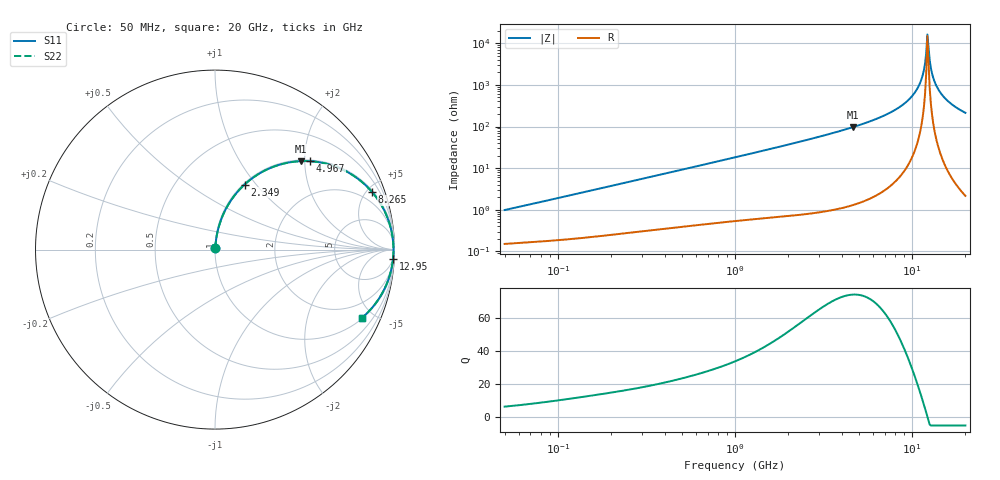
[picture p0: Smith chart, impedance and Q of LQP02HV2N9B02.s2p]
!Murata Part Number: LQP02HV2N9B02
!These Parameters are Measured in Series Mode Connection
!  o--[Z]--o
!Port1  Port2
!  o-------o
!Freq. Start=50[MHz] Stop=20[GHz], 401[Steps]
# Hz S RI R 50
!Freq.(Hz) S11(Real) S11(Imag) S21(Real) S21(Imag) S12(Real) S12(Imag) S22(Real) S22(Imag)
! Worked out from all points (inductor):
!   401 points, 50 MHz to 20 GHz, reference 50 ohm
!   read as one part in series: L = 3.08 nH near 51.52 MHz
!   highest Q = 74.4 at 4.608 GHz (marker M1), where L = 3.32 nH
!   self-resonance near 12.2 GHz
!   S11 on the Smith chart (normalised r, x): 50 MHz: 1.00, +0.02; 2.349 GHz: 1.02, +0.87; 4.967 GHz: 1.03, +2.13; 8.265 GHz: 1.11, +5.43; 12.95 GHz: 5, -38; 20 GHz: 1.04, -4.27
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5e7  0.00161 0.00974  0.9984 -0.00974  0.9984 -0.00974  0.00161 0.00974
1.364002e8  0.00276 0.0257  0.9972 -0.0257  0.9972 -0.0257  0.00276 0.0257
3.721004e8  0.00801 0.0678  0.992 -0.0678  0.992 -0.0678  0.00801 0.0678
1e9  0.0369 0.1744  0.9631 -0.1744  0.9631 -0.1744  0.0369 0.1744
2.348516e9  0.1648 0.3624  0.8352 -0.3624  0.8352 -0.3624  0.1648 0.3624
2.728004e9  0.213 0.4015  0.787 -0.4015  0.787 -0.4015  0.213 0.4015
4.608136e9  0.4802 0.4929  0.5198 -0.4929  0.5198 -0.4929  0.4802 0.4929
4.966507e9  0.5304 0.4924  0.4696 -0.4924  0.4696 -0.4924  0.5304 0.4924
7.442007e9  0.8128 0.3817  0.1872 -0.3817  0.1872 -0.3817  0.8128 0.3817
8.264682e9  0.8759 0.3199  0.1241 -0.3199  0.1241 -0.3199  0.8759 0.3199
9.745021e9  0.9523 0.1985  0.0477 -0.1985  0.0477 -0.1985  0.9523 0.1985
1.082228e10  0.9818 0.1097  0.0182 -0.1097  0.0182 -0.1097  0.9818 0.1097
1.149051e10  0.991 0.0565  0.00899 -0.0565  0.00899 -0.0565  0.991 0.0565
1.183995e10  0.9934 0.0295  0.00655 -0.0295  0.00655 -0.0295  0.9934 0.0295
1.201863e10  0.9941 0.016  0.00589 -0.016  0.00589 -0.016  0.9941 0.016
1.220001e10  0.9944 0.00246  0.0056 -0.00246  0.0056 -0.00246  0.9944 0.00246
1.257102e10  0.9939 -0.0246  0.00612 0.0246  0.00612 0.0246  0.9939 -0.0246
1.295331e10  0.9919 -0.0516  0.00812 0.0516  0.00812 0.0516  0.9919 -0.0516
1.375312e10  0.9835 -0.105  0.0165 0.105  0.0165 0.105  0.9835 -0.105
1.504638e10  0.9603 -0.1822  0.0397 0.1822  0.0397 0.1822  0.9603 -0.1822
1.721783e10  0.9042 -0.2868  0.0958 0.2868  0.0958 0.2868  0.9042 -0.2868
2e10  0.8179 -0.3809  0.1821 0.3809  0.1821 0.3809  0.8179 -0.3809
